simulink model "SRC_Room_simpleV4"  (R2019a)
settings: Solver=ode15s  StartTime=0.0  StopTime=tend  MaxStep=0.1  RelTol=1e-6
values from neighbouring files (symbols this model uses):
  CWlow = split(2)    [Main_Kc_v4.m]
  CWup = split(3)    [Main_Kc_v4.m]
  EHlow = split(4)    [Main_Kc_v4.m]
  EHup = split(5)    [Main_Kc_v4.m]
  HWlow = split(3)    [Main_Kc_v4.m]
  HWup = split(4)    [Main_Kc_v4.m]
  K1 = sign(Kcp(1))    [Main_Kc_v4.m]
  K2 = sign(Kcp(2))    [Main_Kc_v4.m]
  K3 = sign(Kcp(3))    [Main_Kc_v4.m]
  K4 = sign(Kcp(4))    [Main_Kc_v4.m]
  K_amb = 1    [Main_Kc_v4.m]
  K_cw = k(2)    [Main_Kc_v4.m]
  K_eh = k(4)    [Main_Kc_v4.m]
  K_hw = k(3)    [Main_Kc_v4.m]
  K_rw = k(1)    [Main_Kc_v4.m]
  Kc = double(S.Kc)    [SRC_eq_Kc_v3.m]
  Ks1 = vmax/du(1)    [Main_Kc_v4.m]
  Ks2 = vmax/du(2)    [Main_Kc_v4.m]
  Ks3 = vmax/du(3)    [Main_Kc_v4.m]
  Ks4 = vmax/du(4)    [Main_Kc_v4.m]
  Ksu = 1    [Main_Kc_v4.m]
  off1 = -split(2)    [Main_Kc_v4.m]
  off2 = 0    [Main_Kc_v4.m]
  off3 = 0    [Main_Kc_v4.m]
  off4 = -split(4)    [Main_Kc_v4.m]
  RWlow = split(1)    [Main_Kc_v4.m]
  RWup = split(2)    [Main_Kc_v4.m]
  split = split0-split0(3)*ones(1,length(split0))    [Main_Kc_v4.m]    (also in SRC_eq_Kc_v3.m)
  Tamb0 = 18    [Main_Kc_v4.m]
  Tamb1 = 2    [Main_Kc_v4.m]
  Tamb2 = 9    [Main_Kc_v4.m]
  Tamb3 = -5    [Main_Kc_v4.m]
  Tamb4 = -25    [Main_Kc_v4.m]
  Tamb5 = 18    [Main_Kc_v4.m]
  Tamb6 = 5    [Main_Kc_v4.m]
  tau_amb = 15    [Main_Kc_v4.m]
  tau_cw = tau(2)    [Main_Kc_v4.m]
  tau_eh = tau(4)    [Main_Kc_v4.m]
  tau_hw = tau(3)    [Main_Kc_v4.m]
  tau_rw = tau(1)    [Main_Kc_v4.m]
  tauI_sim = max(tauI)    [Main_Kc_v4.m]
  theta_amb = 6    [Main_Kc_v4.m]
  theta_cw = theta(2)    [Main_Kc_v4.m]
  theta_eh = theta(4)    [Main_Kc_v4.m]
  theta_hw = theta(3)    [Main_Kc_v4.m]
  theta_rw = theta(1)    [Main_Kc_v4.m]
  Tr0 = 18    [Main_Kc_v4.m]
  Tsp0 = 18    [Main_Kc_v4.m]
  Tsp1 = 5    [Main_Kc_v4.m]
  Tsp2 = 8    [Main_Kc_v4.m]
  Tsp3 = -Tsp1-Tsp2-2    (= -15)    [Main_Kc_v4.m]
  tTamb1 = 10    [Main_Kc_v4.m]
  tTamb2 = 80    [Main_Kc_v4.m]
  tTamb3 = 140    [Main_Kc_v4.m]
  tTamb4 = 180    [Main_Kc_v4.m]
  tTamb5 = 280    [Main_Kc_v4.m]
  tTamb6 = 350    [Main_Kc_v4.m]
  v10 = 0    [Main_Kc_v4.m]
  v1max = vmax    [Main_Kc_v4.m]
  v1min = 0    [Main_Kc_v4.m]
  v20 = 0    [Main_Kc_v4.m]
  v2max = vmax    [Main_Kc_v4.m]
  v2min = 0    [Main_Kc_v4.m]
  v30 = 0    [Main_Kc_v4.m]
  v3max = vmax    [Main_Kc_v4.m]
  v3min = 0    [Main_Kc_v4.m]
  v40 = 0    [Main_Kc_v4.m]
  v4max = vmax    [Main_Kc_v4.m]
  v4min = 0    [Main_Kc_v4.m]
libraries: simulink x1

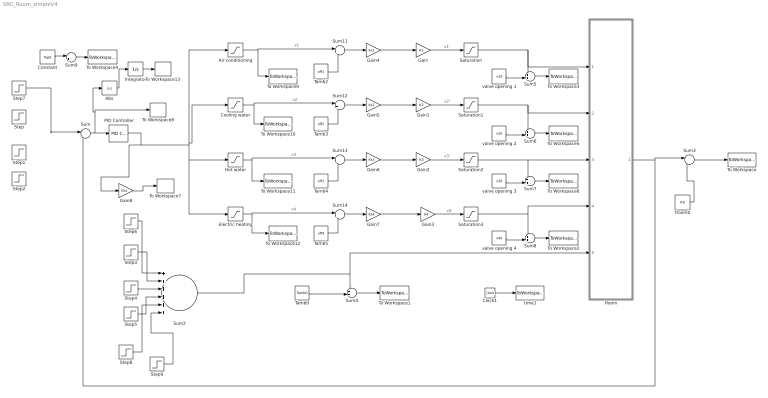
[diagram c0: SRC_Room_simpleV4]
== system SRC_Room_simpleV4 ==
  Abs : Abs
  Air conditioning : Saturate  UpperLimit=RWup  LowerLimit=RWlow
  Clock1 : Clock
  Constant : Constant  Value=Tsp0
  Cooling water : Saturate  UpperLimit=CWup  LowerLimit=CWlow
  Electric heating : Saturate  UpperLimit=EHup  LowerLimit=EHlow
  Gain : Gain  Gain=K1
  Gain1 : Gain  Gain=K2
  Gain2 : Gain  Gain=K3
  Gain3 : Gain  Gain=K4
  Gain4 : Gain  Gain=Ks1
  Gain5 : Gain  Gain=Ks2
  Gain6 : Gain  Gain=Ks3
  Gain7 : Gain  Gain=Ks4
  Gain8 : Gain  Gain=Ksu
  Hot water : Saturate  UpperLimit=HWup  LowerLimit=HWlow
  Integrator : Integrator
  PID Controller : simulink/Continuous/PID Controller  Controller=PI  Form=Parallel  TimeDomain=Continuous-time  SampleTime=-1  IntegratorMethod=Forward Euler  FilterMethod=Forward Euler  ControllerParametersSource=internal  P=Kc  I=Kc/tauI_sim  D=0  UseFilter=on  N=100  TunerSelectOption=Transfer Function Based (PID Tuner App)  InitialConditionSource=internal  InitialConditionForIntegrator=0  InitialConditionForFilter=0  DifferentiatorICPrevScaledInput=0  ExternalReset=none  TrackingMode=off  Kt=1  LimitOutput=on  UpperSaturationLimit=split(5)  LowerSaturationLimit=split(1)  LinearizeAsGain=on  AntiWindupMode=back-calculation  Kb=1  POutMin=[]  POutMax=[]  IOutMin=[]  IOutMax=[]  DOutMin=[]  DOutMax=[]  NOutMin=[]  NOutMax=[]  SumOutMin=[]  SumOutMax=[]  SaturationOutMin=[]  SaturationOutMax=[]  PParamMin=[]  PParamMax=[]  IParamMin=[]  IParamMax=[]  DParamMin=[]  DParamMax=[]  NParamMin=[]  NParamMax=[]  KbParamMin=[]  KbParamMax=[]  KtParamMin=[]  KtParamMax=[]  KbOutMin=[]  KbOutMax=[]  KtOutMin=[]  KtOutMax=[]  IntegratorOutMin=[]  IntegratorOutMax=[]  FilterOutMin=[]  FilterOutMax=[]  SumI1OutMin=[]  SumI1OutMax=[]  SumI2OutMin=[]  SumI2OutMax=[]  SumI3OutMin=[]  SumI3OutMax=[]  SumI4OutMin=[]  SumI4OutMax=[]  SumDOutMin=[]  SumDOutMax=[]  DifferentiatorOutMin=[]  DifferentiatorOutMax=[]  FilterDiffOutCoefMin=[]  FilterDiffOutCoefMax=[]  ReciprocalOutMin=[]  ReciprocalOutMax=[]  SumDenOutMin=[]  SumDenOutMax=[]  SumNumOutMin=[]  SumNumOutMax=[]  DivideOutMin=[]  DivideOutMax=[]  IntegratorContinuousStateAttributes=''  IntegratorStateMustResolveToSignalObject=off  IntegratorRTWStateStorageClass=Auto  FilterContinuousStateAttributes=''  FilterStateMustResolveToSignalObject=off  FilterRTWStateStorageClass=Auto  ParallelPVariant=InternalParameters  IdealPVariant=Disabled  IVariant=InternalParameters  DVariant=Disabled  IntegratorVariant=Continuous  SatVariant=Enabled  AWVariant=BackCalculation  PCopyVariant=Disabled  TRVariant=Disabled  FdbkBlocksVariant=Forward  IdealPFdbkVariant=Disabled  SatFdbkVariant=Disabled  DerivativeFilterVariant=Disabled  NVariant=Disabled  NCopyVariant=Disabled_SignalSpec  FilterICVariant=Disabled  IntegratorICVariant=InternalICs  ExternalResetVariant=Disabled  TRSumVariant=Passthrough  SumFdbkVariant=Disabled  SumVariant=Sum_PI
  Room : Subsystem
  Saturation : Saturate  UpperLimit=v1max  LowerLimit=v1min
  Saturation1 : Saturate  UpperLimit=v2max  LowerLimit=v2min
  Saturation2 : Saturate  UpperLimit=v3max  LowerLimit=v3min
  Saturation3 : Saturate  UpperLimit=v4max  LowerLimit=v4min
  Step : Step  Time=tTamb1  After=Tsp1  SampleTime=0
  Step1 : Step  Time=tTamb2  After=Tsp2  SampleTime=0
  Step2 : Step  Time=tTamb3  After=Tsp3  SampleTime=0
  Step3 : Step  Time=tTamb2  After=Tamb2  SampleTime=0
  Step4 : Step  Time=tTamb3  After=Tamb3  SampleTime=0
  Step5 : Step  Time=tTamb4  After=Tamb4  SampleTime=0
  Step6 : Step  Time=tTamb1  After=Tamb1  SampleTime=0
  Step7 : Step  Time=0  After=0  SampleTime=0
  Step8 : Step  Time=tTamb5  After=Tamb5  SampleTime=0
  Step9 : Step  Time=tTamb6  After=Tamb6  SampleTime=0
  Sum : Sum  Inputs=|+-
  Sum{3,9,11..14} (6 alike) : Sum  Inputs=|++
  Sum2 : Sum  Inputs=++++++
  Sum{4..8} (5 alike) : Sum  Inputs=++|
  Tamb0 : Constant  Value=Tamb0
  Tamb2 : Constant  Value=off1
  Tamb3 : Constant  Value=off2
  Tamb4 : Constant  Value=off3
  Tamb5 : Constant  Value=off4
  To Workspace : ToWorkspace  VariableName=Troom  SampleTime=-1
  To Workspace1 : ToWorkspace  VariableName=Tamb  SampleTime=-1
  To Workspace10 : ToWorkspace  VariableName=v2_pre  SampleTime=-1
  To Workspace11 : ToWorkspace  VariableName=v3_pre  SampleTime=-1
  To Workspace12 : ToWorkspace  VariableName=v4_pre  SampleTime=-1
  To Workspace13 : ToWorkspace  VariableName=IAE  SampleTime=-1
  To Workspace2 : ToWorkspace  VariableName=v4  SampleTime=-1
  To Workspace3 : ToWorkspace  VariableName=v1  SampleTime=-1
  To Workspace4 : ToWorkspace  VariableName=Tsp  SampleTime=-1
  To Workspace5 : ToWorkspace  VariableName=v2  SampleTime=-1
  To Workspace6 : ToWorkspace  VariableName=v3  SampleTime=-1
  To Workspace7 : ToWorkspace  VariableName=u  SampleTime=-1
  To Workspace8 : ToWorkspace  VariableName=e  SampleTime=-1
  To Workspace9 : ToWorkspace  VariableName=v1_pre  SampleTime=-1
  Troom0 : Constant  Value=Tr0
  time1 : ToWorkspace  VariableName=t  SampleTime=-1
  valve opening 1 : Constant  Value=v10
  valve opening 2 : Constant  Value=v20
  valve opening 3 : Constant  Value=v30
  valve opening 4 : Constant  Value=v40
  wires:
  Clock1/1 -> time1/1
  Sum/1 -> Abs/1, To Workspace8/1, PID Controller/1
  Room/1(T) -> Sum/2, Sum3/1  "T"
  Air conditioning/1 -> Sum11/1, To Workspace9/1  "v1"
  Cooling water/1 -> Sum12/1, To Workspace10/1  "v2"
  Hot water/1 -> Sum13/1, To Workspace11/1  "v3"
  Electric heating/1 -> Sum14/1, To Workspace12/1  "v4"
  Step6/1 -> Sum2/1
  Sum2/1 -> Room/5(Tamb), Sum4/1
  Step4/1 -> Sum2/3
  Step3/1 -> Sum2/2
  Step5/1 -> Sum2/4
  Troom0/1 -> Sum3/2
  Sum3/1 -> To Workspace/1
  Tamb0/1 -> Sum4/2
  Sum4/1 -> To Workspace1/1
  Saturation/1 -> Sum5/1, Room/1(vRW)
  Saturation1/1 -> Sum6/1, Room/2(vCW)
  Saturation2/1 -> Sum7/1, Room/3(vHW)
  Saturation3/1 -> Sum8/1, Room/4(vEH)
  valve opening 1/1 -> Sum5/2
  Sum5/1 -> To Workspace3/1
  Sum8/1 -> To Workspace2/1
  Sum6/1 -> To Workspace5/1
  Sum7/1 -> To Workspace6/1
  valve opening 2/1 -> Sum6/2
  valve opening 3/1 -> Sum7/2
  valve opening 4/1 -> Sum8/2
  Sum9/1 -> To Workspace4/1
  Constant/1 -> Sum9/1
  PID Controller/1 -> Gain8/1, Cooling water/1, Air conditioning/1, Electric heating/1, Hot water/1
  Gain/1 -> Saturation/1  "v1'"
  Gain1/1 -> Saturation1/1  "v2'"
  Gain2/1 -> Saturation2/1  "v3'"
  Gain3/1 -> Saturation3/1  "v4'"
  Gain4/1 -> Gain/1
  Sum11/1 -> Gain4/1
  Tamb2/1 -> Sum11/2
  Tamb3/1 -> Sum12/2
  Tamb4/1 -> Sum13/2
  Tamb5/1 -> Sum14/2
  Sum12/1 -> Gain5/1
  Gain5/1 -> Gain1/1
  Sum13/1 -> Gain6/1
  Gain6/1 -> Gain2/1
  Sum14/1 -> Gain7/1
  Gain7/1 -> Gain3/1
  Gain8/1 -> To Workspace7/1
  Integrator/1 -> To Workspace13/1
  Abs/1 -> Integrator/1
  Step8/1 -> Sum2/5
  Step7/1 -> Sum/1
  Step9/1 -> Sum2/6

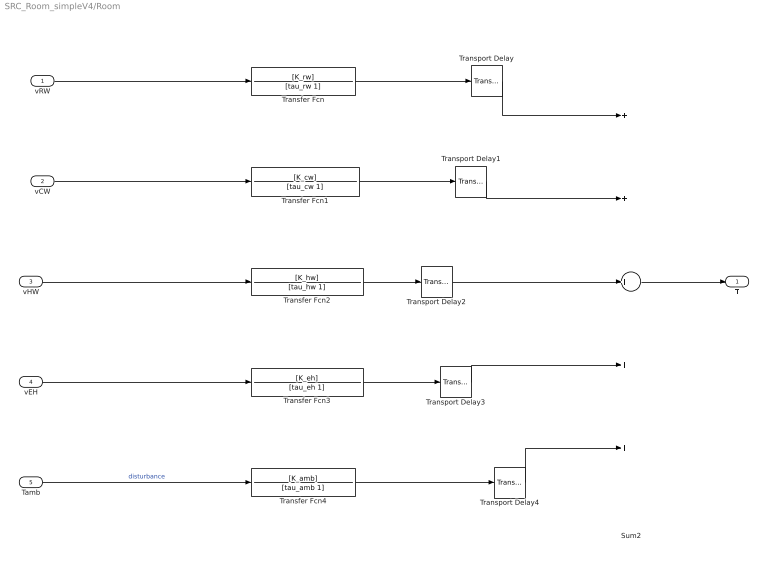
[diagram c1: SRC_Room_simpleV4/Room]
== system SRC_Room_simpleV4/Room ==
  vRW : Inport
  vCW : Inport  Port=2
  vHW : Inport  Port=3
  vEH : Inport  Port=4
  Tamb : Inport  Port=5
  Sum2 : Sum  Inputs=+++++
  Transfer Fcn : TransferFcn  Numerator=[K_rw]  Denominator=[tau_rw 1]
  Transfer Fcn1 : TransferFcn  Numerator=[K_cw]  Denominator=[tau_cw 1]
  Transfer Fcn2 : TransferFcn  Numerator=[K_hw]  Denominator=[tau_hw 1]
  Transfer Fcn3 : TransferFcn  Numerator=[K_eh]  Denominator=[tau_eh 1]
  Transfer Fcn4 : TransferFcn  Numerator=[K_amb]  Denominator=[tau_amb 1]
  Transport Delay : TransportDelay  DelayTime=theta_rw
  Transport Delay1 : TransportDelay  DelayTime=theta_cw
  Transport Delay2 : TransportDelay  DelayTime=theta_hw
  Transport Delay3 : TransportDelay  DelayTime=theta_eh
  Transport Delay4 : TransportDelay  DelayTime=theta_amb
  T : Outport
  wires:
  vRW/1 -> Transfer Fcn/1
  vCW/1 -> Transfer Fcn1/1
  vHW/1 -> Transfer Fcn2/1
  vEH/1 -> Transfer Fcn3/1
  Sum2/1 -> T/1
  Tamb/1 -> Transfer Fcn4/1  "disturbance"
  Transfer Fcn/1 -> Transport Delay/1
  Transfer Fcn1/1 -> Transport Delay1/1
  Transfer Fcn2/1 -> Transport Delay2/1
  Transfer Fcn3/1 -> Transport Delay3/1
  Transfer Fcn4/1 -> Transport Delay4/1
  Transport Delay/1 -> Sum2/1
  Transport Delay1/1 -> Sum2/2
  Transport Delay2/1 -> Sum2/3
  Transport Delay3/1 -> Sum2/4
  Transport Delay4/1 -> Sum2/5
